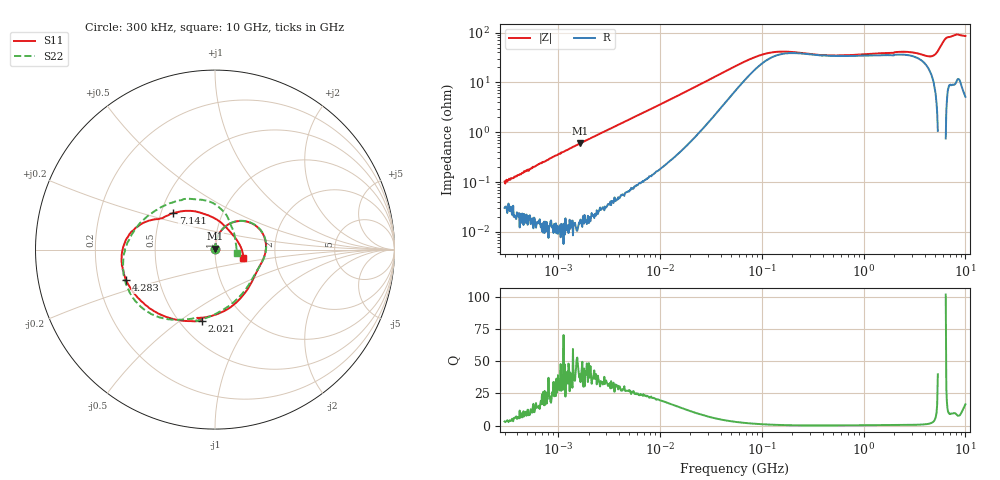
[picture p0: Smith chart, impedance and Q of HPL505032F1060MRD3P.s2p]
! S-Parameter Data Generated by TDK Corporation
! Copyright(C) 2024 TDK Corporation.
! All Rights Reserved.
! TDK P/N: HPL505032F1060MRD3P (SMD / SMT Inductor (Coil))
! Property: L=60nH at 100kHz
! Size(LxWxT): 5x5x3.2mm
! Model Type: s2p (Touchstone File Format Version 1.0)
! Frequency: DC=Yes Start=0.3MHz Stop=10000MHz 802points Log-sweep
! Model Generated on May 28, 2024
! Terms and conditions regarding TDK Simulation Models:
! 1)This simulation model is being provided solely for informational
!  purposes. Please refer to the specifications of the products in
!  terms of detailed characteristics of such products.
! 2)In no event shall TDK Corporation of any of its subsidiaries be
!  liable for any loss or damage arising, directly or indirectly,
!  from any information contained in this simulation model, including,
!  but not limited to loss or damages arising from any inaccuracies,
!  omissions or errors in connection with such information.
! 3)Any and all copyrights on this simulation model are owned by
!  TDK Corporation.  Duplication or redistribution of this simulation
!  model without prior written permission from TDK Corporation
!  is prohibited.
! 4)This simulation model is subject to any modification or change
!  without any prior notice.
! 5)Neither TDK Corporation nor any of its subsidiaries shall make any
!  warranty, express or implied, including but not limited to the
!  correctness, implied warranties of merchantability and fitness for
!  a particular purpose with respect to this simulation models.
! 6)The use of this simulation model shall be deemed to have consented
!  to the terms and conditions hereof.
! Port Assignments:
!  1 ---@@@--- 2
! Applicable Conditions:
!  Temperature = 25 degC
!  DC Bias Current = 0 A
!  Small Signal Operation
# Hz S MA R 50
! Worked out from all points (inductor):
!   801 points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, 300 kHz to 10 GHz, reference 50 ohm
!   read as one part in series: L = 53.2 nH near 318.3 kHz
!   highest Q = 42.4 at 1.667 MHz (marker M1), where L = 57.3 nH
!   S11 on the Smith chart (normalised r, x): 300 kHz: 1.00, +0.00; 2.021 GHz: 0.64, -0.61; 4.283 GHz: 0.32, -0.15; 7.141 GHz: 0.58, +0.26; 10 GHz: 1.37, -0.14
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300000  0.0007559 61.1  0.9998 -0.1  0.9996 -0.0  0.000867 75.6
1666935  0.005414 87.7  0.9998 -0.4  0.9998 -0.4  0.00542 88.0
1713600  0.00555 87.9  0.9999 -0.4  0.9998 -0.4  0.005592 88.5
9671944  0.0312 84.7  0.9977 -2.2  0.9979 -2.2  0.03121 84.7
2.944115e7  0.09687 74.5  0.9805 -6.7  0.9807 -6.7  0.09685 74.6
5.477226e7  0.1776 57.7  0.9242 -11.8  0.9243 -11.8  0.1778 58.0
1.161426e8  0.2766 22.1  0.763 -14.1  0.7631 -14.2  0.2777 22.3
3.126428e8  0.2677 -17.5  0.7294 -10.7  0.7295 -10.7  0.2681 -17.4
8.414386e8  0.2879 -52.0  0.7096 -25.4  0.7097 -25.4  0.2807 -52.9
1.260284e9  0.3294 -73.4  0.663 -37.0  0.6631 -37.0  0.3215 -75.2
1.767019e9  0.3755 -95.5  0.5895 -50.1  0.5896 -50.1  0.3813 -96.8
2.020878e9  0.4034 -100.4  0.5512 -55.5  0.5511 -55.5  0.3959 -105.8
3.050901e9  0.4703 -129.2  0.404 -74.2  0.4039 -74.2  0.4905 -130.2
4.282745e9  0.5244 -161.3  0.2512 -86.0  0.2512 -86.0  0.5307 -157.4
5.040844e9  0.5185 -177.9  0.1854 -83.0  0.1852 -83.1  0.5096 -175.9
5.849356e9  0.459 164.7  0.1539 -67.8  0.1539 -67.8  0.4493 162.7
6.41458e9  0.381 153.9  0.1636 -55.2  0.1637 -55.3  0.3958 146.5
7.141296e9  0.3089 138.6  0.2156 -47.1  0.2158 -47.2  0.3329 124.3
7.875699e9  0.2071 106.7  0.2823 -52.9  0.2824 -52.9  0.2776 100.4
8.658336e9  0.1322 54.5  0.3499 -62.6  0.3501 -62.7  0.2112 74.7
9.105558e9  0.1324 24.2  0.3891 -71.0  0.3897 -71.0  0.1656 58.7
1e10  0.1651 -17.3  0.4384 -89.5  0.4387 -89.6  0.124 -9.9
